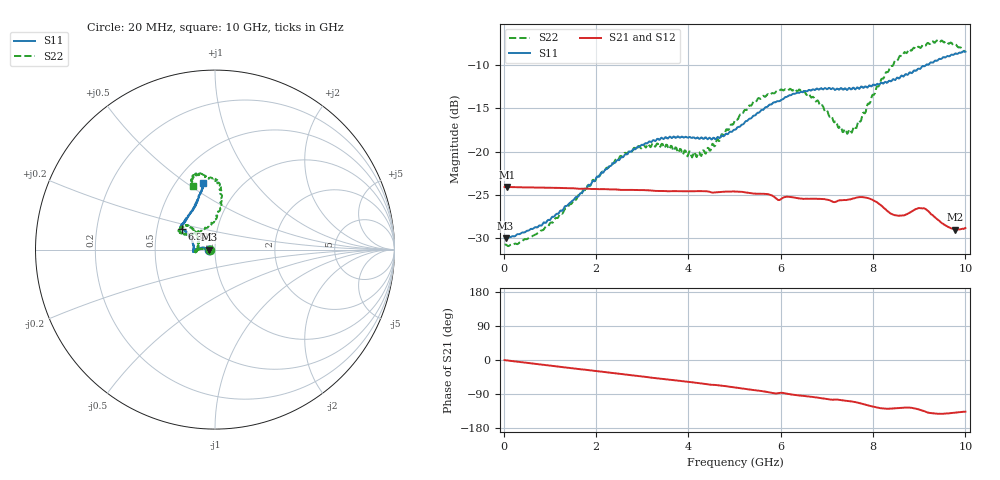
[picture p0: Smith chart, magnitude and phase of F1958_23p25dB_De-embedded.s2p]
! Integrated Device Technology
! Corporate Headquarters
! 6024 Silver Creek Valley Road
! San Jose, CA 95138  USA
! Phone:  1-408-284-8200
! Toll Free:  1-800-223-1366
! Webpage:  http://www.idt.com/
! Timing and RF Division
! 515 Groton Road, Suite 102
! Westford, MA 01886-6024
! Device:  F1958
! Description: 7-bit 0.25 dB Digital Step Attenuator
! Frequency:  0.001 -  6.000 GHz
! Package:  4x4 mm Thin QFN Plastic Package: 24 pin
! Ports:  2 RF, 12 DC
!  Pin  1  = D0
!  Pin  2  = VDD
!  Pin  3  = VMODE
!  Pin  4  = GND
!  Pin  5  = RF1  =  Port 1
!  Pin  6  = GND
!  Pin  7  = GND
!  Pin  8  = GND
!  Pin  9  = GND
!  Pin 10  = GND
!  Pin 11  = GND
!  Pin 12  = GND
!  Pin 13  = GND
!  Pin 14  = RF2  =  Port 2
!  Pin 15  = GND
!  Pin 16  = LE
!  Pin 17  = CLK
!  Pin 18  = DATA
!  Pin 19  = D6
!  Pin 20  = D5
!  Pin 21  = D4
!  Pin 22  = D3
!  Pin 23  = D2
!  Pin 24  = D1
! State:  93
! Atten State:  23.25 dB
! Voltage:  +3.30 Volts
! Current:  0.258 mA
! Data:  The device was measured on a F1958 evaluation board which has
!  individual transmission lines to the RF pins.  Data was collected
!  using a calibrated network analyzer.  The evaluation board was
!  de-embedded using Automatic Fixture Removal (AFR).
!  The reference plane is the edge of the package pin.
! Misc:
!  Action Tracker AT0419
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# GHz S dB R 50
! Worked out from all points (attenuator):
!   500 points, 20 MHz to 10 GHz, reference 50 ohm
!   highest |S21| = -24.09 dB at 80 MHz (marker M1); lowest = -29.0 dB at 9.78 GHz (marker M2)
!   lowest |S11| = -30.0 dB at 40 MHz (marker M3), VSWR 1.07, Z = 46.9 - j0.0417 ohm
!   |S11| at or under -10 dB: start of sweep to 9.149 GHz
!   |S22| runs from -30.9 to -7.2 dB; largest |S21 - S12| = 0.00026
!   S11 on the Smith chart (normalised r, x): 20 MHz: 0.94, -0.00; 6.38 GHz: 0.67, +0.16; 10 GHz: 0.67, +0.58
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0.02  -29.96 -179.0  -24.09 -0.3  -24.09 -0.3  -30.75 -178.8
0.04  -29.99 -179.2  -24.09 -0.6  -24.09 -0.6  -30.72 -178.2
0.08  -29.91 179.4  -24.09 -1.2  -24.09 -1.2  -30.85 -178.4
0.84  -28.39 170.8  -24.16 -12.4  -24.16 -12.4  -29.08 176.3
1.7  -24.76 170.6  -24.28 -24.7  -24.28 -24.7  -24.66 174.7
2.62  -20.38 176.7  -24.41 -37.9  -24.39 -37.9  -20.15 -179.1
3.36  -18.62 -175.9  -24.54 -48.8  -24.54 -48.9  -19.37 -172.0
4.24  -18.55 -179.3  -24.57 -61.1  -24.59 -61.2  -20.08 166.2
4.64  -18.31 171.5  -24.68 -66.6  -24.69 -66.6  -18.59 148.3
5.02  -17.47 160.5  -24.60 -72.7  -24.62 -72.7  -16.29 137.9
5.58  -15.21 150.4  -24.87 -81.8  -24.88 -81.8  -13.82 138.5
6.38  -13.22 148.1  -25.38 -93.4  -25.40 -93.3  -12.96 151.4
6.68  -12.87 146.6  -25.43 -97.3  -25.45 -97.2  -13.74 153.0
7.3  -12.68 140.9  -25.62 -105.8  -25.62 -105.7  -17.08 132.4
7.5  -12.71 138.2  -25.52 -108.7  -25.52 -108.6  -17.44 114.2
7.68  -12.67 135.3  -25.26 -112.8  -25.26 -112.8  -16.48 97.2
7.9  -12.48 129.0  -25.37 -119.9  -25.37 -120.0  -14.45 88.1
8.34  -11.85 119.0  -26.97 -128.7  -26.97 -128.9  -10.67 82.6
8.66  -11.35 113.3  -27.38 -126.1  -27.38 -126.1  -8.68 85.8
9.1  -10.17 107.3  -26.54 -134.7  -26.55 -134.8  -7.71 97.6
9.78  -8.69 100.3  -29.02 -139.0  -29.03 -139.0  -7.65 107.9
10  -8.49 100.0  -28.81 -136.4  -28.85 -136.4  -8.48 109.2
